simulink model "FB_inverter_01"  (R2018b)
settings: Solver=ode23t  StartTime=0.0  StopTime=0.2  MaxStep=1e-5  RelTol=1e-5
libraries: powerlib x23, simulink x2

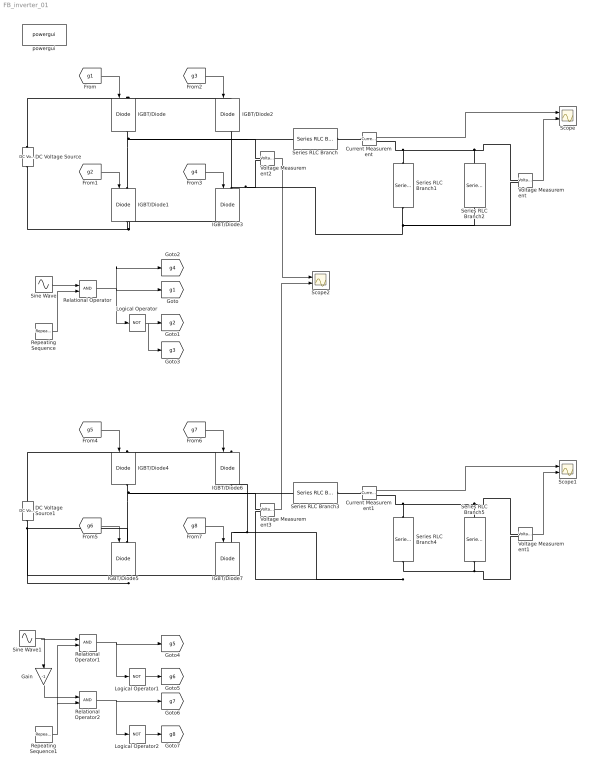
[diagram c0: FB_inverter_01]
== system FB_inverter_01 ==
  Current Measurement : powerlib/Measurements/Current Measurement  PhasorSimulation=off  OutputType=Complex  PSBequivalent=0
  Current Measurement1 : powerlib/Measurements/Current Measurement  PhasorSimulation=off  OutputType=Complex  PSBequivalent=0
  DC Voltage Source : powerlib/Electrical Sources/DC Voltage Source  Amplitude=400  Measurements=None
  DC Voltage Source1 : powerlib/Electrical Sources/DC Voltage Source  Amplitude=400  Measurements=None
  Gain : Gain  Gain=-1
  IGBT/Diode{,1..7} (8 alike) : powerlib/Power Electronics/IGBT//Diode  Ron=1e-3  Rs=1e5  Cs=inf  Measurements=on
  Logical Operator : Logic  Operator=NOT  AllPortsSameDT=off  OutDataTypeStr=boolean
  Logical Operator1 : Logic  Operator=NOT  AllPortsSameDT=off  OutDataTypeStr=boolean
  Logical Operator2 : Logic  Operator=NOT  AllPortsSameDT=off  OutDataTypeStr=boolean
  Relational Operator : RelationalOperator  OutDataTypeStr=boolean  RndMeth=Simplest
  Relational Operator1 : RelationalOperator  OutDataTypeStr=boolean  RndMeth=Simplest
  Relational Operator2 : RelationalOperator  OutDataTypeStr=boolean  RndMeth=Simplest
  Repeating Sequence : simulink/Sources/Repeating Sequence  rep_seq_t=[0 0.0001 0.0002]  rep_seq_y=[-400 400 -400]
  Repeating Sequence1 : simulink/Sources/Repeating Sequence  rep_seq_t=[0 0.0001 0.0002]  rep_seq_y=[-400 400 -400]
  Scope : Scope  NumInputPorts=2
  Scope1 : Scope  NumInputPorts=2
  Scope2 : Scope  NumInputPorts=2
  Series RLC Branch : powerlib/Elements/Series RLC Branch  LConnTagsString=__new0  RConnTagsString=__new0  BranchType=L  Resistance=1  Inductance=1e-3  SetiL0=off  InitialCurrent=0  Capacitance=1e-6  Setx0=off  InitialVoltage=0  Measurements=None
  Series RLC Branch1 : powerlib/Elements/Series RLC Branch  LConnTagsString=__new0  RConnTagsString=__new0  BranchType=C  Resistance=1  Inductance=1e-3  SetiL0=off  InitialCurrent=0  Capacitance=47e-6  Setx0=off  InitialVoltage=0  Measurements=None
  Series RLC Branch2 : powerlib/Elements/Series RLC Branch  LConnTagsString=__new0  RConnTagsString=__new0  BranchType=R  Resistance=5  Inductance=1e-3  SetiL0=off  InitialCurrent=0  Capacitance=100e-6  Setx0=off  InitialVoltage=0  Measurements=None
  Series RLC Branch3 : powerlib/Elements/Series RLC Branch  LConnTagsString=__new0  RConnTagsString=__new0  BranchType=L  Resistance=1  Inductance=1e-3  SetiL0=off  InitialCurrent=0  Capacitance=1e-6  Setx0=off  InitialVoltage=0  Measurements=None
  Series RLC Branch4 : powerlib/Elements/Series RLC Branch  LConnTagsString=__new0  RConnTagsString=__new0  BranchType=C  Resistance=1  Inductance=1e-3  SetiL0=off  InitialCurrent=0  Capacitance=47e-6  Setx0=off  InitialVoltage=0  Measurements=None
  Series RLC Branch5 : powerlib/Elements/Series RLC Branch  LConnTagsString=__new0  RConnTagsString=__new0  BranchType=R  Resistance=5  Inductance=1e-3  SetiL0=off  InitialCurrent=0  Capacitance=100e-6  Setx0=off  InitialVoltage=0  Measurements=None
  Sine Wave : Sin  Amplitude=300  Frequency=2*pi*10  SampleTime=0
  Sine Wave1 : Sin  Amplitude=300  Frequency=2*pi*10  SampleTime=0
  Voltage Measurement{,1..3} (4 alike) : powerlib/Measurements/Voltage Measurement  PhasorSimulation=off  OutputType=Complex  PSBequivalent=0
  powergui : powerlib/powergui  Priority=1  SimulationMode=Continuous  SampleTime=50e-6  frequency=60  Iterations=50  frequencyindice=0  Pbase=100e6  ErrMax=1e-4  UnitsV=kV  UnitsW=MW  buscounter=0  FunctionMessages=on  echomessages=on  EnableUseOfTLC=off  CurrentSourceSwitches=on  DisableSnubberDevices=on  DisableRonSwitches=on  DisableVfSwitches=on  DisplayEquations=off  SolverType=Tustin/Backward Euler (TBE)  Interpol=off  ExternalGateDelay=off  methode=off  Ts=100  x0status=blocks  SPID=on  SwTol=0  HookPort=off  RestoreLinks=warning  ResistiveCurrentMeasurement=off  Frange=[0:2:500]  Ylog=off  Xlog=on  ShowGrid=off  save=off  variable=ZData  structure=0  ZoomFFT=off  StartTime=0.0  cycles=1  DisplayStyle=1  fundamental=60  FreqAxis=off  MaxFrequency=1000  frequencyindicesteady=1  RmsSteady=1  display=off
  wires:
  [g4] -> IGBT/Diode3/1
  [g2] -> IGBT/Diode1/1
  [g1] -> IGBT/Diode/1
  [g3] -> IGBT/Diode2/1
  Repeating Sequence/1 -> Relational Operator/2
  Sine Wave/1 -> Relational Operator/1
  Relational Operator/1 -> Logical Operator/1, [g4], [g1]
  Logical Operator/1 -> [g3], [g2]
  Current Measurement/1 -> Scope/1
  Voltage Measurement/1 -> Scope/2
  Voltage Measurement1/1 -> Scope1/2
  Current Measurement1/1 -> Scope1/1
  Logical Operator1/1 -> [g6]
  Relational Operator1/1 -> [g5], Logical Operator1/1
  Sine Wave1/1 -> Gain/1, Relational Operator1/1
  Repeating Sequence1/1 -> Relational Operator2/2, Relational Operator1/2
  [g7] -> IGBT/Diode6/1
  [g5] -> IGBT/Diode4/1
  [g6] -> IGBT/Diode5/1
  [g8] -> IGBT/Diode7/1
  Gain/1 -> Relational Operator2/1
  Relational Operator2/1 -> Logical Operator2/1, [g7]
  Logical Operator2/1 -> [g8]
  Voltage Measurement2/1 -> Scope2/1
  Voltage Measurement3/1 -> Scope2/2
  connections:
  IGBT/Diode1/LConn1 -- Voltage Measurement2/LConn1 -- Series RLC Branch/LConn1 -- IGBT/Diode/RConn1
  DC Voltage Source/RConn1 -- IGBT/Diode2/LConn1 -- IGBT/Diode/LConn1
  IGBT/Diode1/RConn1 -- DC Voltage Source/LConn1 -- IGBT/Diode3/RConn1
  IGBT/Diode3/LConn1 -- Voltage Measurement2/LConn2 -- Series RLC Branch2/RConn1 -- Voltage Measurement/LConn2 -- Series RLC Branch1/RConn1 -- IGBT/Diode2/RConn1
  Series RLC Branch1/LConn1 -- Current Measurement/RConn1 -- Series RLC Branch2/LConn1 -- Voltage Measurement/LConn1
  Series RLC Branch/RConn1 -- Current Measurement/LConn1
  IGBT/Diode5/LConn1 -- Voltage Measurement3/LConn1 -- Series RLC Branch3/LConn1 -- IGBT/Diode4/RConn1
  IGBT/Diode6/LConn1 -- IGBT/Diode4/LConn1 -- DC Voltage Source1/RConn1
  DC Voltage Source1/LConn1 -- IGBT/Diode5/RConn1 -- IGBT/Diode7/RConn1
  Series RLC Branch5/RConn1 -- Voltage Measurement1/LConn2 -- Voltage Measurement3/LConn2 -- IGBT/Diode7/LConn1 -- IGBT/Diode6/RConn1 -- Series RLC Branch4/RConn1
  Series RLC Branch4/LConn1 -- Current Measurement1/RConn1 -- Voltage Measurement1/LConn1 -- Series RLC Branch5/LConn1
  Series RLC Branch3/RConn1 -- Current Measurement1/LConn1
